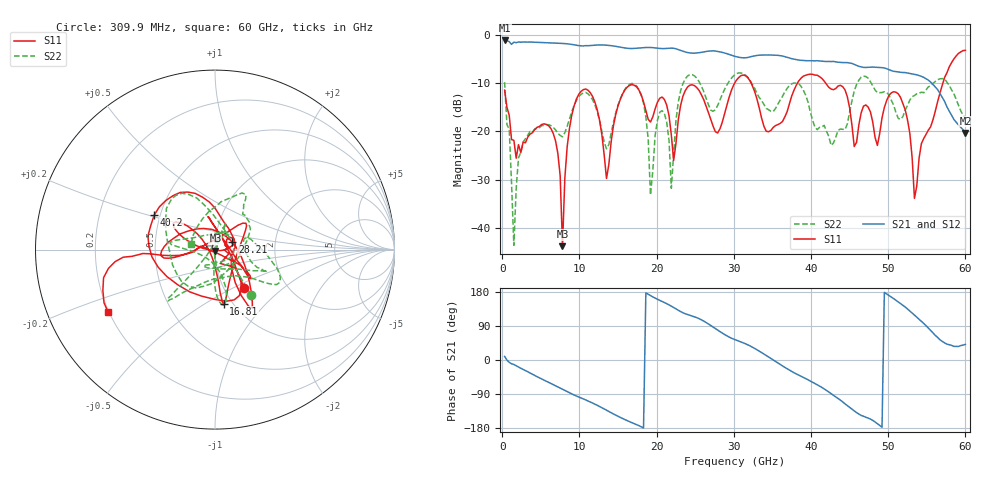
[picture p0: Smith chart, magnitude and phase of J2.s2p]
!Keysight Technologies,N5227A,US51270214,A.10.65.11
!Date: Thursday, October 15, 2020 07:41:48
!Correction: S11(Full 2 Port(1,2))
!S21(Full 2 Port(1,2))
!S12(Full 2 Port(1,2))
!S22(Full 2 Port(1,2))
!S2P File: Measurements: S11, S21, S12, S22:
# Hz S  dB  R 50
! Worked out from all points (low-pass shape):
!   200 points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, 309.9 MHz to 60 GHz, reference 50 ohm
!   highest |S21| = -1.18 dB at 309.9 MHz (marker M1); lowest = -20.3 dB at 60 GHz (marker M2)
!   |S21| within 3 dB of the highest: start of sweep to 29.59 GHz
!   lowest |S11| = -43.8 dB at 7.809 GHz (marker M3), VSWR 1.01, Z = 50.3 - j0.596 ohm
!   |S11| at or under -10 dB: start of sweep to 30.12 GHz; 32.23 GHz to 38.25 GHz (6.022 GHz wide, 17.1 % of centre); 41.89 GHz to 57.09 GHz (15.2 GHz wide, 30.7 % of centre)
!   |S22| runs from -43.6 to -7.9 dB; largest |S21 - S12| = 0.12
!   S11 on the Smith chart (normalised r, x): 309.9 MHz: 1.24, -0.57; 16.81 GHz: 0.91, -0.60; 28.21 GHz: 1.21, +0.11; 40.2 GHz: 0.46, +0.21; 60 GHz: 0.20, -0.26
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3.0995e8  -11.46 -52.6  -1.18 9.5  -1.78 16.8  -9.82 -51.5
1.50975e9  -21.87 -16.8  -1.53 -11.8  -1.37 -10.9  -43.62 154.2
2.70955e9  -22.26 30.9  -1.50 -24.8  -1.45 -24.6  -22.20 71.3
6.6089e9  -20.44 12.1  -1.71 -65.0  -1.70 -64.9  -19.19 62.8
7.8087e9  -43.79 -66.6  -1.80 -77.1  -1.78 -77.1  -21.14 107.5
8.70855e9  -19.43 167.9  -1.92 -86.4  -1.93 -86.5  -17.48 150.0
1.050825e10  -11.38 149.6  -2.31 -102.5  -2.29 -102.8  -12.08 170.2
1.350775e10  -29.77 -168.1  -2.16 -132.5  -2.16 -132.5  -23.63 -129.4
1.68072e10  -10.33 -81.0  -2.85 -165.5  -2.86 -165.5  -10.09 -81.4
1.92068e10  -18.08 -14.3  -2.64 170.0  -2.65 170.0  -33.17 -81.8
2.04066e10  -13.15 36.9  -2.83 157.5  -2.84 157.5  -16.06 68.2
2.190635e10  -20.73 61.6  -2.76 142.1  -2.78 142.1  -31.78 112.5
2.370605e10  -11.60 -169.4  -3.56 122.1  -3.57 122.1  -9.16 -133.6
2.82053e10  -19.50 23.9  -3.55 74.9  -3.54 75.0  -13.51 -45.2
3.030495e10  -9.49 -52.2  -4.54 52.5  -4.55 52.6  -8.08 -29.7
3.450425e10  -20.08 -11.8  -4.18 7.9  -4.19 7.8  -15.52 17.7
4.02033e10  -8.19 150.3  -5.38 -58.7  -5.40 -58.9  -17.72 -56.5
4.56024e10  -23.15 5.0  -6.13 -134.8  -6.13 -134.5  -11.65 104.3
5.010165e10  -12.57 -38.9  -7.23 170.0  -7.24 170.6  -12.49 -115.5
5.22013e10  -15.53 -31.8  -7.83 139.9  -7.86 139.9  -15.62 7.5
5.34011e10  -33.89 -65.8  -8.21 118.7  -8.21 118.6  -12.60 35.8
6e10  -3.22 -149.8  -20.33 41.3  -20.32 41.5  -17.25 167.4
